|Texas Instruments Incorporated
| Universal Microphone to 2VRMS Analog input, 24-Bit, 192 kHz Stereo Front-End
| Marketing part#   Digital Voltage Range   Package-type   #pins
| PCM1860   1.62V-3.6V   TSSOP   30
| PCM1861   1.62V-3.6V   TSSOP   30
| PCM1862   1.62V-3.6V   TSSOP   30
| PCM1863   1.62V-3.6V   TSSOP   30
| PCM1864   1.62V-3.6V   TSSOP   30
| PCM1865   1.62V-3.6V   TSSOP   30
[IBIS Ver]   4.1
[File name]   pcm186x.ibs
[File Rev]   1.0
[Date]   2/17/2014
[Source]
| Texas Instruments Incorporated.
| Analog-eLab Design Center, HPA
| 12500 TI Blvd
| Dallas, TX -75243
[Notes]   Revision History:
| Rev 1.0: 2/17/2014
| - Initial version of the model
| - Model generated from simulations in TISPICE
| - Model matched to SPICE simulation
| - C_comp although listed in numerical order of value are
|   obtained from varying PVT conditions. For PVT conditions for
|   each specific value refer the buffer description under
|   respective [Model]. IBIS model user is responsible for using
|   appropriate C_comp to simulate for Signal Integrity.
| - Combined Pulldown/up non-monotonicity warnings for INOUT models
|   reflect simulation results and can be safely ignored.
|*EXCEPTION:   *
|* - For GPIO and SDA models,There will be small leakage currents in   *
|* - POWER clamp IV-table because of the resistor (RES3T_NWELL) connected   *
|* - to the pad.   *
[Disclaimer]
| This model is designed as an aid for customers of Texas Instruments.
| TI and its licensors and suppliers make no warranties, either expressed
| or implied, with respect to this  model, including the warranties of
| merchantability or fitness for a particular purpose. The model is
| provided solely on an "as is" basis. The entire risk as to its quality
| and performance is with the customer.
[Copyright]
(C) Copyright 2014 Texas Instruments Incorporated.All rights reserved.
|   PCM1860DBT
[Component]   PCM1860DBT
[Manufacturer]   TI
[Package]   |30 TSSOP  -  DBT package
|   typ   min   max
R_pkg   0.09881   0.06258   0.12678
L_pkg   2.46532nH   1.97125nH   3.78535nH
C_pkg   0.28986pF   0.21539pF   0.50145pF
[Pin]  signal_name   model_name   R_pin   L_pin   C_pin
1   VINL2/VIN1M   NC   0.14960   4.08088nH  0.51680pF
2   VINR2/VIN2M   NC   0.14576   3.45299nH  0.40652pF
3   VINL1/VIN1P   NC   0.14023   2.76524nH  0.26820pF
4   VINR1/VIN2P   NC   0.11243   2.31697nH  0.22996pF
5   Mic_Bias   NC   0.08753   1.99724nH  0.21980pF
6   VREF   NC   0.04823   1.66984nH  0.25634pF
7   AGND   GND   0.03559   1.65500nH  0.26490pF
8   AVDD   POWER   0.03623   1.60458nH  0.27042pF
9   DVDD   POWER   0.09007   2.02781nH  0.21886pF
10   IOVDD   POWER   0.08541   1.97051nH  0.21614pF
11   DGND   GND   0.08636   1.98436nH  0.21795pF
12   LDO   NC   0.03847   1.73024nH  0.27179pF
13   XO   xo   0.06258   2.13329nH  0.28531pF
14   XI   xi   0.12376   3.16969nH  0.39140pF
15   SCKI   INPUT   0.12678   3.78535nH  0.50145pF
16   LRCK   INOUT   0.12223   3.72675nH  0.50045pF
17   BCK   INOUT   0.11929   3.11199nH  0.38915pF
18   DOUT   INOUT   0.10814   2.35068nH  0.24563pF
19   INT   GPIO   0.09398   2.08412nH  0.21768pF
20   MD6   GPIO   0.08546   1.97276nH  0.21677pF
21   MD5   GPIO   0.08548   1.97125nH  0.21539pF
22   MD4   GPIO   0.08776   1.99910nH  0.21630pF
23   DOUT2/MD2   SDA   0.08648   1.98317nH  0.21542pF
24   MD3   INPUT   0.08887   2.01292nH  0.21741pF
25   MD1   INPUT   0.09206   2.05281nH  0.22030pF
26   MD0   INPUT   0.10053   2.16066nH  0.22532pF
27   VINL4/VIN4M   NC   0.11243   2.31697nH  0.22894pF
28   VINR4/VIN3M   NC   0.14023   2.76524nH  0.26805pF
29   VINL3/VIN4P   NC   0.14576   3.45299nH  0.40649pF
30   VINR3/VIN3P   NC   0.14960   4.08088nH  0.51679pF
|   PCM1861DBT
[Component]   PCM1861DBT
[Manufacturer]   TI
[Package]   |30 TSSOP  -  DBT package
|   typ   min   max
R_pkg   0.09494   0.06258   0.12678
L_pkg   2.44304nH   1.97125nH   3.78535nH
C_pkg   0.29221pF   0.21539pF   0.50235pF
[Pin]  signal_name   model_name   R_pin   L_pin   C_pin
1   VINL2/VIN1M   NC   0.14960   4.08088nH  0.51680pF
2   VINR2/VIN2M   NC   0.14576   3.45299nH  0.40652pF
3   VINL1/VIN1P   NC   0.14023   2.76524nH  0.26820pF
4   VINR1/VIN2P   NC   0.11243   2.31697nH  0.22996pF
5   Mic_Bias   NC   0.08753   1.99724nH  0.21980pF
6   VREF   NC   0.04823   1.66984nH  0.25634pF
7   AGND   GND   0.03559   1.65500nH  0.26490pF
8   AVDD   POWER   0.03623   1.60458nH  0.27042pF
9   DVDD   POWER   0.09007   2.02781nH  0.21886pF
10   IOVDD   POWER   0.08541   1.97051nH  0.21614pF
11   DGND   GND   0.08636   1.98436nH  0.21795pF
12   LDO   NC   0.03847   1.73024nH  0.27192pF
13   XO   xo   0.06258   2.13329nH  0.28764pF
14   XI   xi   0.06948   2.85769nH  0.42114pF
15   SCKI   INPUT   0.12678   3.78535nH  0.50235pF
16   LRCK   INOUT   0.12223   3.72675nH  0.50046pF
17   BCK   INOUT   0.11929   3.11199nH  0.38915pF
18   DOUT   INOUT   0.10814   2.35068nH  0.24563pF
19   INT   GPIO   0.09398   2.08412nH  0.21768pF
20   MD6   GPIO   0.08546   1.97276nH  0.21677pF
21   MD5   GPIO   0.08548   1.97125nH  0.21539pF
22   MD4   GPIO   0.08776   1.99910nH  0.21630pF
23   DOUT2/MD2   SDA   0.08648   1.98317nH  0.21542pF
24   MD3   INPUT   0.08887   2.01292nH  0.21741pF
25   MD1   INPUT   0.09206   2.05281nH  0.22030pF
26   MD0   INPUT   0.10053   2.16066nH  0.22533pF
27   VINL4/VIN4M   NC   0.11243   2.31697nH  0.22894pF
28   VINR4/VIN3M   NC   0.14023   2.76524nH  0.26805pF
29   VINL3/VIN4P   NC   0.14576   3.45299nH  0.40649pF
30   VINR3/VIN3P   NC   0.14960   4.08088nH  0.51679pF
|   PCM1862DBT
[Component]   PCM1862DBT
[Manufacturer]   TI
[Package]   |30 TSSOP  -  DBT package
|   typ   min   max
R_pkg   0.09504   0.06258   0.12678
L_pkg   2.44547nH   1.97125nH   3.78535nH
C_pkg   0.29241pF   0.21540pF   0.50358pF
[Pin]  signal_name   model_name   R_pin   L_pin   C_pin
1   VINL2/VIN1M   NC   0.14960   4.08088nH  0.51680pF
2   VINR2/VIN2M   NC   0.14576   3.45299nH  0.40652pF
3   VINL1/VIN1P   NC   0.14023   2.76524nH  0.26820pF
4   VINR1/VIN2P   NC   0.11243   2.31697nH  0.22996pF
5   Mic_Bias   NC   0.08753   1.99724nH  0.21980pF
6   VREF   NC   0.04823   1.66984nH  0.25634pF
7   AGND   GND   0.03559   1.65500nH  0.26490pF
8   AVDD   POWER   0.03623   1.60458nH  0.27042pF
9   DVDD   POWER   0.09007   2.02781nH  0.21886pF
10   IOVDD   POWER   0.08541   1.97051nH  0.21614pF
11   DGND   GND   0.08636   1.98436nH  0.21795pF
12   LDO   NC   0.03847   1.73024nH  0.27188pF
13   XO   xo   0.06258   2.13329nH  0.28661pF
14   XI   xi   0.07091   2.89176nH  0.42368pF
15   SCKI   INPUT   0.12678   3.78535nH  0.50358pF
16   LRCK   INOUT   0.12223   3.72675nH  0.50047pF
17   BCK   INOUT   0.11929   3.11199nH  0.38916pF
18   DOUT   INOUT   0.10814   2.35068nH  0.24563pF
19   GPIO3/INTC   GPIO   0.09398   2.08412nH  0.21768pF
20   GPIO2/INTB/DMCLK   GPIO   0.08546   1.97276nH  0.21677pF
21   GPIO1/INT-A/DMIN   GPIO   0.08548   1.97125nH  0.21540pF
22   MISO/GPIO0MD4   GPIO   0.08776   1.99910nH  0.21630pF
23   MOSI/SDA   SDA   0.08648   1.98317nH  0.21543pF
24   MC/SCL   INPUT   0.08887   2.01292nH  0.21741pF
25   MS/AD   INPUT   0.09206   2.05281nH  0.22030pF
26   MD0   INPUT   0.10053   2.16066nH  0.22532pF
27   VINL4/VIN4M   NC   0.11243   2.31697nH  0.22894pF
28   VINR4/VIN3M   NC   0.14023   2.76524nH  0.26805pF
29   VINL3/VIN4P   NC   0.14576   3.45299nH  0.40649pF
30   VINR3/VIN3P   NC   0.14960   4.08088nH  0.51679pF
|   PCM1863DBT
[Component]   PCM1863DBT
[Manufacturer]   TI
[Package]   |30 TSSOP  -  DBT package
|   typ   min   max
R_pkg   0.09371   0.05229   0.12678
L_pkg   2.44086nH   1.97125nH   3.78535nH
C_pkg   0.29378pF   0.21539pF   0.50403pF
[Pin]  signal_name   model_name   R_pin   L_pin   C_pin
1   VINL2/VIN1M   NC   0.14960   4.08088nH  0.51680pF
2   VINR2/VIN2M   NC   0.14576   3.45299nH  0.40652pF
3   VINL1/VIN1P   NC   0.14023   2.76524nH  0.26820pF
4   VINR1/VIN2P   NC   0.11243   2.31697nH  0.22996pF
5   Mic_Bias   NC   0.08753   1.99724nH  0.21980pF
6   VREF   NC   0.04823   1.66984nH  0.25634pF
7   AGND   GND   0.03559   1.65500nH  0.26490pF
8   AVDD   POWER   0.03623   1.60458nH  0.27042pF
9   DVDD   POWER   0.09007   2.02781nH  0.21886pF
10   IOVDD   POWER   0.08541   1.97051nH  0.21614pF
11   DGND   GND   0.08636   1.98436nH  0.21795pF
12   LDO   NC   0.03847   1.73024nH  0.27197pF
13   XO   xo   0.06258   2.13329nH  0.28833pF
14   XI   xi   0.05229   2.82716nH  0.44063pF
15   SCKI   INPUT   0.12678   3.78535nH  0.50403pF
16   LRCK   INOUT   0.12223   3.72675nH  0.50048pF
17   BCK   INOUT   0.11929   3.11199nH  0.38916pF
18   DOUT   INOUT   0.10814   2.35068nH  0.24563pF
19   GPIO3/INTC   GPIO   0.09398   2.08412nH  0.21768pF
20   GPIO2/INTB/DMCLK   GPIO   0.08546   1.97276nH  0.21677pF
21   GPIO1/INT-A/DMIN   GPIO   0.08548   1.97125nH  0.21539pF
22   MISO/GPIO0MD4   GPIO   0.08776   1.99910nH  0.21630pF
23   MOSI/SDA   SDA   0.08648   1.98317nH  0.21542pF
24   MC/SCL   INPUT   0.08887   2.01292nH  0.21741pF
25   MS/AD   INPUT   0.09206   2.05281nH  0.22030pF
26   MD0   INPUT   0.10053   2.16066nH  0.22533pF
27   VINL4/VIN4M   NC   0.11243   2.31697nH  0.22894pF
28   VINR4/VIN3M   NC   0.14023   2.76524nH  0.26805pF
29   VINL3/VIN4P   NC   0.14576   3.45299nH  0.40649pF
30   VINR3/VIN3P   NC   0.14960   4.08088nH  0.51679pF
|   PCM1864DBT
[Component]   PCM1864DBT
[Manufacturer]   TI
[Package]   |30 TSSOP  -  DBT package
|   typ   min   max
R_pkg   0.09504   0.06258   0.12678
L_pkg   2.44547nH   1.97125nH   3.78535nH
C_pkg   0.29241pF   0.21540pF   0.50358pF
[Pin]  signal_name   model_name   R_pin   L_pin   C_pin
1   VINL2/VIN1M   NC   0.14960   4.08088nH  0.51680pF
2   VINR2/VIN2M   NC   0.14576   3.45299nH  0.40652pF
3   VINL1/VIN1P   NC   0.14023   2.76524nH  0.26820pF
4   VINR1/VIN2P   NC   0.11243   2.31697nH  0.22996pF
5   Mic_Bias   NC   0.08753   1.99724nH  0.21980pF
6   VREF   NC   0.04823   1.66984nH  0.25634pF
7   AGND   GND   0.03559   1.65500nH  0.26490pF
8   AVDD   POWER   0.03623   1.60458nH  0.27042pF
9   DVDD   POWER   0.09007   2.02781nH  0.21886pF
10   IOVDD   POWER   0.08541   1.97051nH  0.21614pF
11   DGND   GND   0.08636   1.98436nH  0.21795pF
12   LDO   NC   0.03847   1.73024nH  0.27188pF
13   XO   xo   0.06258   2.13329nH  0.28661pF
14   XI   xi   0.07091   2.89176nH  0.42368pF
15   SCKI   INPUT   0.12678   3.78535nH  0.50358pF
16   LRCK   INOUT   0.12223   3.72675nH  0.50047pF
17   BCK   INOUT   0.11929   3.11199nH  0.38916pF
18   DOUT   INOUT   0.10814   2.35068nH  0.24563pF
19   GPIO3/INTC   GPIO   0.09398   2.08412nH  0.21768pF
20   GPIO2/INTB/DMCLK   GPIO   0.08546   1.97276nH  0.21677pF
21   GPIO1/INT-A/DMIN   GPIO   0.08548   1.97125nH  0.21540pF
22   MISO/GPIO0MD4   GPIO   0.08776   1.99910nH  0.21630pF
23   MOSI/SDA   SDA   0.08648   1.98317nH  0.21543pF
24   MC/SCL   INPUT   0.08887   2.01292nH  0.21741pF
25   MS/AD   INPUT   0.09206   2.05281nH  0.22030pF
26   MD0   INPUT   0.10053   2.16066nH  0.22532pF
27   VINL4/VIN4M   NC   0.11243   2.31697nH  0.22894pF
28   VINR4/VIN3M   NC   0.14023   2.76524nH  0.26805pF
29   VINL3/VIN4P   NC   0.14960   4.08088nH  0.51679pF
|   PCM1865DBT
[Component]   PCM1865DBT
[Manufacturer]   TI
[Package]   |30 TSSOP  -  DBT package
|   typ   min   max
R_pkg   0.09371   0.05229   0.12678
L_pkg   2.44086nH   1.97125nH   3.78535nH
C_pkg   0.29378pF   0.21539pF   0.50403pF
[Pin]  signal_name   model_name   R_pin   L_pin   C_pin
1   VINL2/VIN1M   NC   0.14960   4.08088nH  0.51680pF
2   VINR2/VIN2M   NC   0.14576   3.45299nH  0.40652pF
3   VINL1/VIN1P   NC   0.14023   2.76524nH  0.26820pF
4   VINR1/VIN2P   NC   0.11243   2.31697nH  0.22996pF
5   Mic_Bias   NC   0.08753   1.99724nH  0.21980pF
6   VREF   NC   0.04823   1.66984nH  0.25634pF
7   AGND   GND   0.03559   1.65500nH  0.26490pF
8   AVDD   POWER   0.03623   1.60458nH  0.27042pF
9   DVDD   POWER   0.09007   2.02781nH  0.21886pF
10   IOVDD   POWER   0.08541   1.97051nH  0.21614pF
11   DGND   GND   0.08636   1.98436nH  0.21795pF
12   LDO   NC   0.03847   1.73024nH  0.27197pF
13   XO   xo   0.06258   2.13329nH  0.28833pF
14   XI   xi   0.05229   2.82716nH  0.44063pF
15   SCKI   INPUT   0.12678   3.78535nH  0.50403pF
16   LRCK   INOUT   0.12223   3.72675nH  0.50048pF
17   BCK   INOUT   0.11929   3.11199nH  0.38916pF
18   DOUT   INOUT   0.10814   2.35068nH  0.24563pF
19   GPIO3/INTC   GPIO   0.09398   2.08412nH  0.21768pF
20   GPIO2/INTB/DMCLK   GPIO   0.08546   1.97276nH  0.21677pF
21   GPIO1/INT-A/DMIN   GPIO   0.08548   1.97125nH  0.21539pF
22   MISO/GPIO0MD4   GPIO   0.08776   1.99910nH  0.21630pF
23   MOSI/SDA   SDA   0.08648   1.98317nH  0.21542pF
24   MC/SCL   INPUT   0.08887   2.01292nH  0.21741pF
25   MS/AD   INPUT   0.09206   2.05281nH  0.22030pF
26   MD0   INPUT   0.10053   2.16066nH  0.22533pF
27   VINL4/VIN4M   NC   0.11243   2.31697nH  0.22894pF
28   VINR4/VIN3M   NC   0.14023   2.76524nH  0.26805pF
29   VINL3/VIN4P   NC   0.14576   3.45299nH  0.40649pF
30   VINR3/VIN3P   NC   0.14960   4.08088nH  0.51679pF
|   Model Selectors
[Model Selector] INPUT
input_1p8   1.8V  digital input
input_3p3   3.3V  digital input
[Model Selector] INOUT
inout_1p8   1.8V  digital I/O
inout_3p3   3.3V  digital I/O
[Model Selector] GPIO
gpio_1p8   1.8V  digital I/O
gpio_3p3   3.3V  digital I/O
[Model Selector] SDA
sda_1p8   1.8V  digital I/O_open_drain
sda_3p3   3.3V  digital I/O_open_drain
| Models and submodels in the file (10): input_1p8 (Input), input_3p3 (Input), xi (Input), xo (Output), inout_1p8 (I/O), inout_3p3 (I/O), gpio_1p8 (I/O), gpio_3p3 (I/O), sda_1p8 (I/O_open_drain), sda_3p3 (I/O_open_drain)
